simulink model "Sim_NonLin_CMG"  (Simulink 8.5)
settings: Solver=ode4  StartTime=0.0  StopTime=3600*3  FixedStep=Ts*5  RelTol=1e-3
InitFcn:
  | start
StopFcn:
  | Pl3
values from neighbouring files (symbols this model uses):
  com_dir = com_dir/sqrt(com_dir'*com_dir)    [start.m]    (also in start1.m; start2.m; start3.m)
  d2r = pi/180    (= 0.0174532925199)    [start.m]    (also in start1.m; start2.m; start3.m; Dead_Band_DF.m)
  ini = [wbo; atto; Hco]    [start.m]    (also in start1.m; start2.m; start3.m)
  J = [0.119416e9, -0.476e7,   -0.1216e7;     -0.476e7,     0.40408e8, -0.30121e6;     -0.1216e7,   -0.30121e6,  0.110166e9]    [start.m]    (also in start1.m; start2.m; start3.m)
  KshC = 2*Wdot_Lim_CMG/WlimC    [start.m]    (also in start1.m; start2.m; start3.m)
  nt = 12    [start.m]    (also in start1.m; start2.m; start3.m)
  omg = 20*wo    (= 0.022)    [start.m]    (also in start1.m; start2.m; start3.m)
  r2d = 180/pi    (= 57.2957795131)    [start.m]    (also in start1.m; start2.m; start3.m)
  thecmd = 20    [start.m]    (also in start1.m = 0.1; start2.m; start3.m)
  Wdot_Lim_CMG = 0.0001*d2r    (= 1.74532925199e-06)    [start.m]    (also in start1.m; start2.m; start3.m)
  Wlim_CMG = 0.01*d2r    (= 0.000174532925199)    [start.m]    (also in start1.m; start2.m; start3.m)
  wo = 0.0011    [start.m]    (also in start1.m; start2.m; start3.m)
  zeb = 0.95    [start.m]    (also in start1.m; start2.m; start3.m)
undefined symbols (not defined in the file or in its folder): Rigbod_Dynam_LVLH, Torq_Lim, Wlim

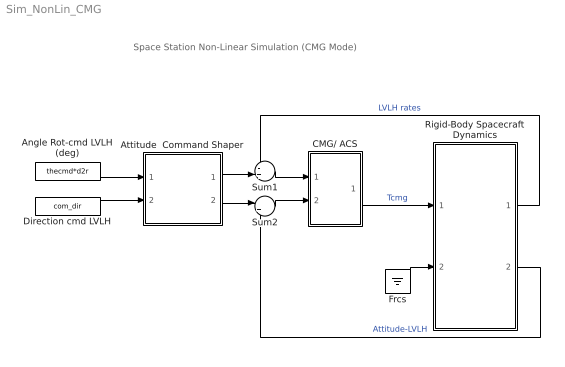
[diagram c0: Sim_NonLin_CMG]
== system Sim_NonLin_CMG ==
  note: Space Station Non-Linear Simulation (CMG Mode)
  Angle Rot-cmd LVLH (deg) : Constant  Value=thecmd*d2r
  Attitude  Command Shaper : Subsystem
  CMG/ ACS : Subsystem
  Direction cmd LVLH : Constant  Value=com_dir
  Frcs : Ground
  Rigid-Body Spacecraft Dynamics : Subsystem
  Sum1 : Sum  Inputs=-+|
  Sum2 : Sum  Inputs=|+-
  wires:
  Rigid-Body Spacecraft Dynamics/2(atti-lv) -> Sum2/2  "Attitude-LVLH"
  Sum2/1 -> CMG/ ACS/2(ater)
  Rigid-Body Spacecraft Dynamics/1(w-lv) -> Sum1/1  "LVLH rates"
  Direction cmd LVLH/1 -> Attitude  Command Shaper/2(dir)
  Angle Rot-cmd LVLH (deg)/1 -> Attitude  Command Shaper/1(cmd)
  Sum1/1 -> CMG/ ACS/1(wl)
  CMG/ ACS/1(Tq) -> Rigid-Body Spacecraft Dynamics/1(Tcmg)  "Tcmg"
  Frcs/1 -> Rigid-Body Spacecraft Dynamics/2(f(i))
  Attitude  Command Shaper/2(att-cmd) -> Sum2/1
  Attitude  Command Shaper/1(w-cmd) -> Sum1/2

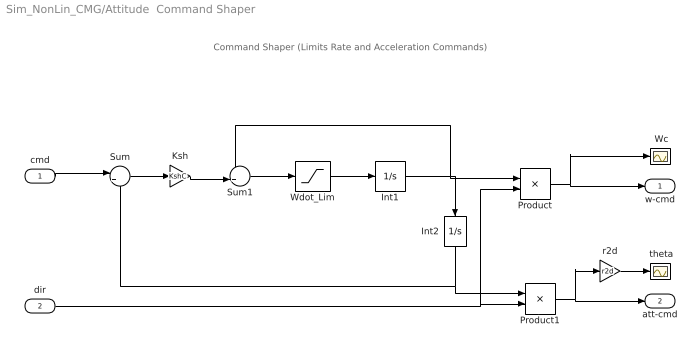
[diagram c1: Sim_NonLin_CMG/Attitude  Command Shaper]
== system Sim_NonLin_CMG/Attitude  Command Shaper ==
  note: Command Shaper (Limits Rate and Acceleration Commands)
  cmd : Inport  PortDimensions=1
  dir : Inport  Port=2  PortDimensions=3
  " Wc" : Scope
  " theta" : Scope
  Int1 : Integrator  LimitOutput=on  UpperSaturationLimit=Wlim_CMG  LowerSaturationLimit=-Wlim_CMG
  Int2 : Integrator  UpperSaturationLimit=Wlim  LowerSaturationLimit=-Wlim
  Ksh : Gain  Gain=KshC
  Product : Product
  Product1 : Product
  Sum : Sum  Inputs=|+-
  Sum1 : Sum  Inputs=-+|
  Wdot_Lim : Saturate  UpperLimit=Wdot_Lim_CMG  LowerLimit=-Wdot_Lim_CMG
  r2d : Gain  Gain=r2d
  w-cmd : Outport  PortDimensions=3
  att-cmd : Outport  Port=2  PortDimensions=3
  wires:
  Wdot_Lim/1 -> Int1/1
  Sum1/1 -> Wdot_Lim/1
  Int1/1 -> Product/1, Sum1/1, Int2/1
  Sum/1 -> Ksh/1
  Ksh/1 -> Sum1/2
  Int2/1 -> Sum/2, Product1/1
  cmd/1 -> Sum/1
  dir/1 -> Product/2, Product1/2
  r2d/1 -> " theta"/1
  Product/1 -> w-cmd/1, " Wc"/1
  Product1/1 -> att-cmd/1, r2d/1

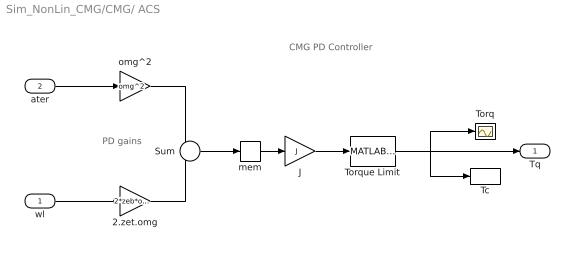
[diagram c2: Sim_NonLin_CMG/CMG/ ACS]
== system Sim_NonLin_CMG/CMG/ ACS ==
  note: CMG PD Controller
  note: PD gains
  wl : Inport
  ater : Inport  Port=2  PortDimensions=3
  2.zet.omg : Gain  Gain=2*zeb*omg
  J : Gain  Gain=J  Multiplication=Matrix(K*u)
  Sum : Sum  Inputs=--
  Tc : ToWorkspace  VariableName=Tcmg  SampleTime=-1
  Torq : Scope
  Torque Limit : MATLABFcn  MATLABFcn=Torq_Lim( u(1:3) )  OutputDimensions=3
  mem : Memory
  omg^2 : Gain  Gain=omg^2
  Tq : Outport
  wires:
  wl/1 -> 2.zet.omg/1
  Sum/1 -> mem/1
  2.zet.omg/1 -> Sum/2
  ater/1 -> omg^2/1
  omg^2/1 -> Sum/1
  J/1 -> Torque Limit/1
  mem/1 -> J/1
  Torque Limit/1 -> Tq/1, Torq/1, Tc/1

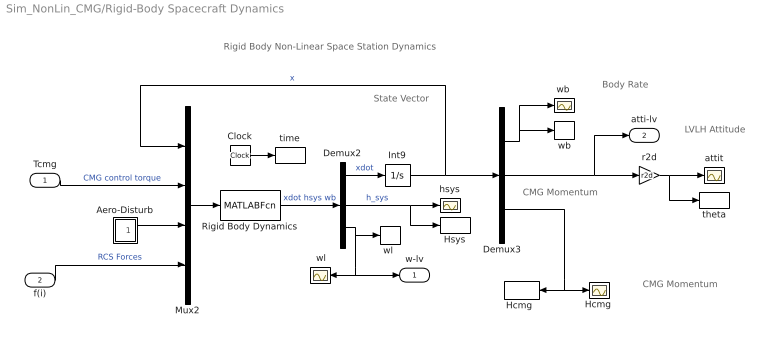
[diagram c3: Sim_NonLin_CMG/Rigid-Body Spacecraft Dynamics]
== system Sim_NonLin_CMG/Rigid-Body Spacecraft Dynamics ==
  note: Rigid Body Non-Linear Space Station Dynamics
  note: CMG Momentum
  note: LVLH Attitude
  note: Body Rate
  note: CMG Momentum
  note: State Vector
  Tcmg : Inport  PortDimensions=3
  f(i) : Inport  Port=2  PortDimensions=nt
  " wl" : Scope
  Aero-Disturb : Subsystem
  Clock : Clock
  Demux2 : Demux  Outputs=[9,3,3]
  Demux3 : Demux  Outputs=[3,3,3]
  "Hcmg " : Scope
  "Hcmg  " : ToWorkspace  VariableName=Hcmg  SampleTime=-1
  Hsys : ToWorkspace  VariableName=Hsys  SampleTime=-1
  Int9 : Integrator  InitialCondition=ini
  Mux2 : Mux  Inputs=[9, 3, 3, nt]
  Rigid Body Dynamics : MATLABFcn  MATLABFcn=Rigbod_Dynam_LVLH( u(1:9), u(10:12), u(13:15), u(16:15+nt) )  OutputDimensions=15
  attit : Scope
  hsys : Scope
  r2d : Gain  Gain=r2d
  theta : ToWorkspace  VariableName=theta  SampleTime=-1
  time : ToWorkspace  VariableName=time  SampleTime=-1
  wb : ToWorkspace  VariableName=wb  SampleTime=-1
  "wb " : Scope
  "wl " : ToWorkspace  VariableName=wl  SampleTime=-1
  w-lv : Outport
  atti-lv : Outport  Port=2
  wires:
  Rigid Body Dynamics/1 -> Demux2/1  "xdot hsys wb"
  Demux2/1 -> Int9/1  "xdot"
  Int9/1 -> Demux3/1, Mux2/1  "x"
  Tcmg/1 -> Mux2/2  "CMG control torque"
  Demux2/3 -> "wl "/1, w-lv/1, " wl"/1
  Demux2/2 -> hsys/1, Hsys/1  "h_sys"
  Demux3/2 -> r2d/1, atti-lv/1
  Demux3/3 -> "Hcmg  "/1, "Hcmg "/1
  f(i)/1 -> Mux2/4  "RCS Forces"
  r2d/1 -> attit/1, theta/1
  Clock/1 -> time/1
  Mux2/1 -> Rigid Body Dynamics/1
  Demux3/1 -> "wb "/1, wb/1
  Aero-Disturb/1(Td) -> Mux2/3

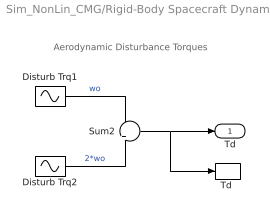
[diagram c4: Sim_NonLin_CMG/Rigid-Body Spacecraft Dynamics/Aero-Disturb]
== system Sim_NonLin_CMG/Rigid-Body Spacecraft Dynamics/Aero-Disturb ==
  note: Aerodynamic Disturbance Torques
  Disturb Trq1 : Sin  Amplitude=[1, 3, 1]  Bias="[1  8  1]"  Frequency=[wo, wo, wo]  SampleTime=0
  Disturb Trq2 : Sin  Amplitude=[1, 1, 1]*0.5  Frequency=[wo, wo, wo]*2  SampleTime=0
  Sum2 : Sum  Inputs=+|+
  "Td " : ToWorkspace  VariableName=Td  SampleTime=-1
  Td : Outport
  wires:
  Disturb Trq1/1 -> Sum2/1  "wo"
  Sum2/1 -> Td/1, "Td "/1
  Disturb Trq2/1 -> Sum2/2  "2*wo"
